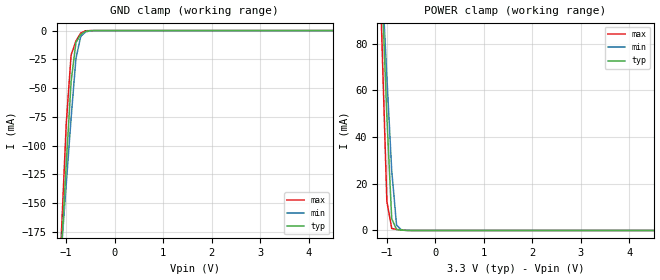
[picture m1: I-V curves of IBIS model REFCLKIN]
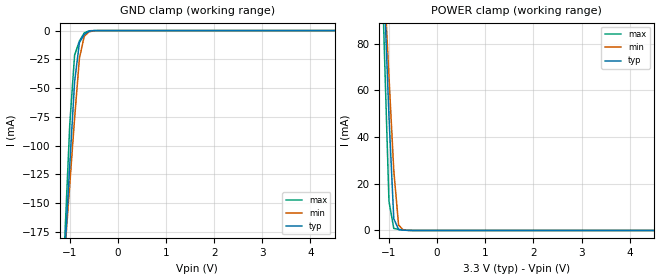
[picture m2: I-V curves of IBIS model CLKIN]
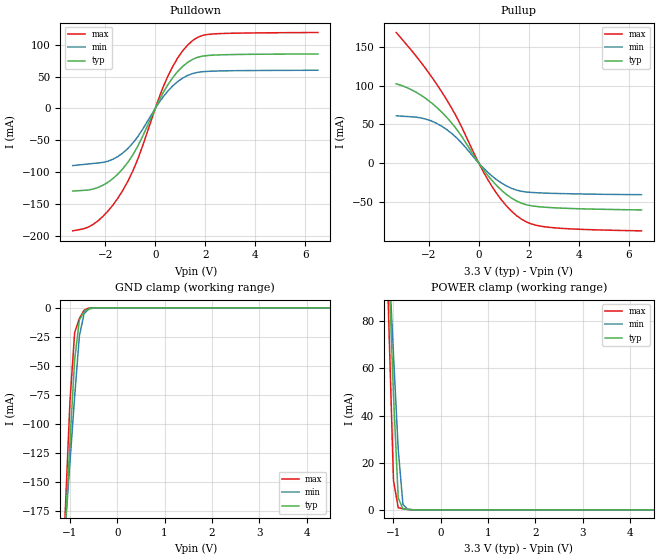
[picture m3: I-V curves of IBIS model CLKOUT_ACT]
|   Texas Instruments Incorporated
|   Data Transmissions Products
|   IBIS Model for CDCF5801A & CDC5801A Clock Multiplier
|   24 pin SSOP Package (DBQ)
[IBIS Ver]   3.2
[Comment char]   |_char
[File name]   cdc5801a.ibs
[File Rev]   1.6
[Date]   07-10-2003
[Source]   File originated at Texas Instruments Incorporated.
|Revision log:
|  1.3, 2004-01-22: Added Vmeas, Cref, Rref, Vref to CLKOUT
|   Corrected Vinl,Vinh for REFCLKIN to VDDREF/2 +/-0.2V
|  1.4, 2004-01-26: updated GND and POWER clamp characteristics to
|   33C10 CDC family clamp characteristics.
|   removed non-monotinic waring on pullup / pulldown plots
|  1.6  2004-01-29: Added models for POWER-DOWN and STOPB conditions of
|   clock output pair.
[Notes]
| All clamp structures used for that design are referenced to VDDO!
| Please take care to update Vinl, Vinh for REFCLKIN and CLKIN to your
| application settings of VDDREF and VDDPD !
| EXAMPLES ARE:
| Vinl = 0.4V   |set this value to VDDREF/2-0.2V, value shown is for VDDREF=1.2V
| Vinh = 0.8V   |set this value to VDDREF/2+0.2V, value shown is for VDDREF=1.2V
| Vinl = 1.3V   |set this value to VDDREF/2-0.2V, value shown is for VDDREF=3.0V
| Vinh = 2.0V   |set this value to VDDREF/2+0.2V, value shown is for VDDREF=3.6V
| . . . . . . . . . . . . . . . . . . . . . . . . . . . . . . . . . . . . . . .
| Vinl = 0.43V   |set this value to VDDPD*0.3, value shown at VDDPD=1.44V (+20%)
| Vinh = 0.84V   |set this value to VDDPD*0.7, value shown at VDDPD=1.2V
| Vinl = 1.08V   |set this value to VDDPD*0.3, value shown at VDDPD=3.6V
| Vinh = 2.10V   |set this value to VDDPD*0.7, value shown at VDDPD=3.0V
[Disclaimer]
|(C) Copyright Texas Instruments Incorporated 1998
|   All rights reserved
|  Texas Instruments Incorporated hereby grants the user of this IBIS
| model a non-exclusive, nontransferable license to use this IBIS model
| under the following terms.  Before using this IBIS model, the user
| should read this license.  If the user does not accept these terms,
| the IBIS model should be returned to Texas Instruments within 30 days.
|   The user is granted this license only to use the IBIS model and
| is not granted rights to sell, load, rent, lease or license the IBIS
| model in whole or in part, or in modified form to anyone other than
| user.  User may modify the IBIS model to suit its specific applications
| but rights to derivative works and such modifications shall belong to
| Texas Instruments.
|   This IBIS model is provided on an "AS IS" basis and Texas Instruments
| makes absolutely no warranty with respect to the information contained
| herein.  TEXAS INSTRUMENTS DISCLAIMS AND CUSTOMER WAIVES ALL WARRANTIES,
| EXPRESS OR IMPLIED, INCLUDING WARRANTIES OF MERCHANTABILITY OR FITNESS
| FOR A PARTICULAR PURPOSE. The entire risk as to quality and performance
| is with the Customer. ACCORDINGLY, IN NO EVENT SHALL THE COMPANY BE LIABLE
| FOR ANY DAMAGES, WHETHER IN CONTRACT OR TORT,INCLUDING ANY LOST PROFITS
| OR OTHER INCIDENTAL, CONSEQUENTIAL, EXEMPLARY, OR PUNITIVE DAMAGES ARISING
| OUT OF THE USE OR APPLICATION OF THE IBIS model provided in this package.
| Further, Texas Instruments reserves the right to discontinue or make changes
| without notice to any product herein to improve reliability, function, or
| design. Texas Instruments does not convey any license under patent rights
| or any other intellectual property rights, including those of third parties.
[Copyright]   Copyright 2001, Texas Instruments, All Rights Reserved
[Component]   CDCF5801
[Manufacturer]  Texas Instruments Incorporated
[Package]   | SSOP, 24-pin DBQ
|   typ   min   max
R_pkg   0.0446   0.0410   0.0495
L_pkg   3.522n   3.22n   4.05n
C_pkg   0.134p   0.084p   0.245p
[Pin]   signal_name   model_name   R_pin   L_pin   C_pin
   1   VDDREF   POWER   0.0413   3.93n   0.239p
   2   REFCLK   REFCLKIN   0.0397   3.57n   0.149p
   3   VDDP   POWER   0.0417   3.77n   0.152p
   4   GNDP   GND   0.0470   3.43n   0.093p
   5   GND   GND   0.0463   3.33n   0.087p
   6   LEADLAG   CLKIN   0.0495   3.35n   0.088p
   7   DLYCTRL   CLKIN   0.0463   3.22n   0.084p
   8   GNDPA   GND   0.0474   3.28n   0.086p
   9   VDDPA   POWER   0.0474   3.29n   0.094p
   10   VDDPD   POWER   0.0413   3.57n   0.142p
   11   STOPB   CLKIN   0.0411   3.61n   0.150p
   12   PWRDNB   CRTLIN   0.0452   4.05n   0.245p
   13   P2   CRTLIN   0.0430   3.97n   0.240p
   14   MULTI1   CRTLIN   0.0413   3.62n   0.150p
   15   MULTI0   CRTLIN   0.0410   3.68n   0.148p
   16   VDDO   POWER   0.0477   3.36n   0.097p
   17   GNDO   GND   0.0474   3.02n   0.087p
   18   CLKOUTB   CLKOUT   0.0477   3.27n   0.084p
   19   NC   NC   0.0478   3.27n   0.084p
   20   CLKOUT   CLKOUT   0.0473   3.30n   0.087p
   21   GNDO   GND   0.0477   3.35n   0.097p
   22   VDDO   POWER   0.0410   3.68n   0.148p
   23   P1   CRTLIN   0.0413   3.62n   0.150p
   24   P0   CRTLIN   0.0429   3.98n   0.241p
[Diff_pin]   inv_pin   vdiff   tdelay_typ   tdelay_min   tdelay_max
| The '+' pin is Diff_pin and the '-' pin is the inv_pin
20   18   0   0 0 0
[Model Selector]   CLKOUT
CLKOUT_ACT   clock pair normal operation, outputs active or 3-state
CLKOUT_PWRDWN  clock pair in POWER DOWN mode
CLKOUT_STOPB   clock pair in STOPB mode
| Models and submodels in the file (6): REFCLKIN (Input), CLKIN (Input), CRTLIN (Input), CLKOUT_ACT (3-state), CLKOUT_PWRDWN (Terminator), CLKOUT_STOPB (Terminator)
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|   REFCLK INPUT
[Model]   REFCLKIN
Model_type   Input
Vinl = 1.45V   |set this value to VDDREF/2-0.2V, value shown is for VDDREF=3.3V
Vinh = 1.85V   |set this value to VDDREF/2+0.2V, value shown is for VDDREF=3.3V
Polarity   Non-Inverting
|Signals   REFCLK
|variable   typ   min   max
C_comp   1.9pF   NA   NA
[Temperature Range] 25.0   0   85.0
[Voltage range]   3.3V   3.135V   3.465V
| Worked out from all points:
|   GND clamp passes 1 mA (typ) near -0.62 V on its own axis
|   POWER clamp passes 1 mA (typ) near -0.81 V on its own axis
[GND Clamp]
|   40C:3.3V:nominal   85C:3.135V:weak   0C:3.465V:strong
|   Voltage   I(typ)   I(min)   I(max)
-3.6V     -2.067A    -1.637A    -2.608A
-1.1V     -191.2mA   -191.4mA   -177mA
-1V       -116.4mA   -133.6mA   -81.31mA
-900mV    -44.54mA   -76.34mA   -21.33mA
-800mV    -10.43mA   -24.19mA   -9.069mA
-700mV    -3.354mA   -4.946mA   -2.091mA
-600mV    -584uA     -1.128mA   -168.8uA
-400mV    -2.829uA   -16.92uA   -75.16nA
6.6V      809.2pA    1.216nA    1.067nA
[POWER Clamp]
|   40C:3.3V:nominal   85C:3.135V:weak   0C:3.465V:strong
|   Voltage   I(typ)   I(min)   I(max)
-3.6V     1.449A     1.143A     1.831A
-1.2V     156.3mA    148.7mA    150.2mA
-1.1V     102.5mA    107.3mA    80.16mA
-1V       48.84mA    65.9mA     12.51mA
-900mV    5.043mA    25.68mA    873.6uA
-800mV    395.6uA    2.294mA    462.2uA
-700mV    140.4uA    201.9uA    209.5uA
6.6V      -652.1pA   -3.956nA   -915pA
|   CLOCK INPUT   *
[Model]   CLKIN
Model_type   Input
Vinl = 1.08V
Vinh = 2.1V
Polarity   Non-Inverting
|Signals   Stopb, DlyCtrl, LeadLag
|variable   typ   min   max
C_comp   1.9pF   NA   NA
[Temperature Range] 25.0   0   85.0
[Voltage range]   3.3V   3.135V   3.465V
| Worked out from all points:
|   GND clamp passes 1 mA (typ) near -0.62 V on its own axis
|   POWER clamp passes 1 mA (typ) near -0.81 V on its own axis
[GND Clamp]
|   40C:3.3V:nominal   85C:3.0V:weak   0C:3.6V:strong
|   Voltage   I(typ)   I(min)   I(max)
-3.6V     -2.067A    -1.637A    -2.608A
-1.1V     -191.2mA   -191.4mA   -177mA
-1V       -116.4mA   -133.6mA   -81.31mA
-900mV    -44.54mA   -76.34mA   -21.33mA
-800mV    -10.43mA   -24.19mA   -9.069mA
-700mV    -3.354mA   -4.946mA   -2.091mA
-600mV    -584uA     -1.128mA   -168.8uA
-400mV    -2.829uA   -16.92uA   -75.16nA
6.6V      809.2pA    1.216nA    1.067nA
[POWER Clamp]
|   40C:3.3V:nominal   85C:3.0V:weak   0C:3.6V:strong
|   Voltage   I(typ)   I(min)   I(max)
-3.6V     1.449A     1.143A     1.831A
-1.2V     156.3mA    148.7mA    150.2mA
-1.1V     102.5mA    107.3mA    80.16mA
-1V       48.84mA    65.9mA     12.51mA
-900mV    5.043mA    25.68mA    873.6uA
-800mV    395.6uA    2.294mA    462.2uA
-700mV    140.4uA    201.9uA    209.5uA
6.6V      -652.1pA   -3.956nA   -915pA
|   Clock Output  MODEL
[Model]   CLKOUT_ACT
Model_type   3-state
Polarity   Non-Inverting
|Signals   CLKOUT,CLKOUTB
Vmeas = 1.65V   |Vox used for timing measurements (nom crosspoint voltage)
|   at typical VDD=3.3V and typical model. Note that real cross
|   point may off by +/-200mV
Cref = 0pF   |load capacitance for timing spec (to ground!)
Rref = 50   |50 ohms to Vocm in differential configuration (100ohms
|   channel to channel).
Vref = 1.51V   |Vref equals to output common mode voltage (Vocm) of the
|   differential pair at typical VDD=3.3V and typical model.
|variable   typ   min   max
C_comp   2.9pF   NA   NA
[Temperature Range] 25.0   0   85.0
[Voltage range]   3.3V   3.135V   3.465V
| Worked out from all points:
|   slope of the pulldown table from 0 to 0.495 V, typ, clamps not added: 13.4 ohm
|   slope of the pullup table from 0 to 0.495 V, typ, clamps not added: 23.4 ohm
|   GND clamp passes 1 mA (typ) near -0.62 V on its own axis
|   POWER clamp passes 1 mA (typ) near -0.81 V on its own axis
[Pullup]
|   40C:3.3V:nominal   85C:3.0V:weak   0C:3.6V:strong
|   Voltage   I(typ)   I(min)   I(max)
-3.3V     102.2mA    61.1mA     168.3mA
-2.7V     94.74mA    59.75mA    145.5mA
-2.3V     87.33mA    58.28mA    129.3mA
-1.5V     66.35mA    48mA       92.77mA
-900mV    44.26mA    33.06mA    60.19mA
-100mV    4.824mA    3.653mA    6.428mA
500mV     -21.26mA   -15.83mA   -28.61mA
1.1V      -40.14mA   -29.19mA   -54.84mA
1.5V      -48.55mA   -34.54mA   -67.28mA
2.1V      -54.84mA   -37.63mA   -78.2mA
2.7V      -56.8mA    -38.54mA   -82.13mA
6.5V      -60.14mA   -40.52mA   -87.1mA
[Pulldown]
|   40C:3.3V:nominal   85C:3.0V:weak   0C:3.6V:strong
|   Voltage   I(typ)   I(min)   I(max)
-3.3V     -130mA     -89.98mA   -192.6mA
-2.7V     -128.5mA   -87.54mA   -187.1mA
-2.3V     -124.6mA   -85.9mA    -177.2mA
-1.7V     -110.6mA   -80.17mA   -152.4mA
-1.3V     -95.04mA   -70.25mA   -129.1mA
-700mV    -59.56mA   -44.58mA   -80mA
100mV     8.405mA    6.18mA     11.41mA
500mV     37.03mA    27.08mA    50.39mA
900mV     58.18mA    42.19mA    79.53mA
1.5V      77.18mA    54.85mA    106.8mA
2.3V      83.68mA    58.52mA    117mA
6.5V      85.57mA    59.94mA    119.3mA
[GND Clamp]
|   40C:3.3V:nominal   85C:3.0V:weak   0C:3.6V:strong
|   Voltage   I(typ)   I(min)   I(max)
-3.6V     -2.067A    -1.637A    -2.608A
-1.1V     -191.2mA   -191.4mA   -177mA
-1V       -116.4mA   -133.6mA   -81.31mA
-900mV    -44.54mA   -76.34mA   -21.33mA
-800mV    -10.43mA   -24.19mA   -9.069mA
-700mV    -3.354mA   -4.946mA   -2.091mA
-600mV    -584uA     -1.128mA   -168.8uA
-400mV    -2.829uA   -16.92uA   -75.16nA
6.6V      809.2pA    1.216nA    1.067nA
[POWER Clamp]
|   40C:3.3V:nominal   85C:3.0V:weak   0C:3.6V:strong
|   Voltage   I(typ)   I(min)   I(max)
-3.6V     1.449A     1.143A     1.831A
-1.2V     156.3mA    148.7mA    150.2mA
-1.1V     102.5mA    107.3mA    80.16mA
-1V       48.84mA    65.9mA     12.51mA
-900mV    5.043mA    25.68mA    873.6uA
-800mV    395.6uA    2.294mA    462.2uA
-700mV    140.4uA    201.9uA    209.5uA
6.6V      -652.1pA   -3.956nA   -915pA
[ramp]
| variable   typ   min   max
dV/dt_r   1.3349E+00/2.3464E-10  1.0383E+00/3.2360E-10  1.6105E+00/1.5531E-10
dV/dt_f   1.5716E+00/2.7330E-10  1.2940E+00/3.9326E-10  1.8255E+00/1.4306E-10
